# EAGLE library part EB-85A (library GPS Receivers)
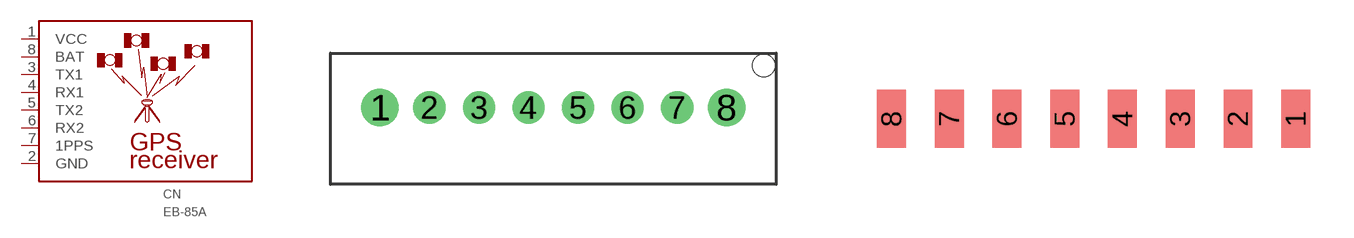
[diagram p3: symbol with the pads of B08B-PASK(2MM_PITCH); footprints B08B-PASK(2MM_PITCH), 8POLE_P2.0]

Designator prefix CN

## EB-85A-PASK  [B08B-PASK(2MM_PITCH)]
1  VCC
2  GND
3  TX1
4  RX1
5  TX2
6  RX2
7  1PPS
8  BAT

## EB-85A-PAD_P2.0  [8POLE_P2.0]
Pads as for B08B-PASK(2MM_PITCH)

## Footprint B08B-PASK(2MM_PITCH) (pad centres in mm)
B08B-PASK _PA series 2.0mm pitch connector Producted by JST.
drill 1: 1 -7,0; 8 7,0
drill 0.8: 2 -5,0; 3 -3,0; 4 -1,0; 5 1,0; 6 3,0; 7 5,0
hole 0.9 at 8.5,1.7

## Footprint 8POLE_P2.0 (pad centres in mm)
smd 1 x 2: 1 7,0; 2 5,0; 3 3,0; 4 1,0; 5 -1,0; 6 -3,0; 7 -5,0; 8 -7,0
